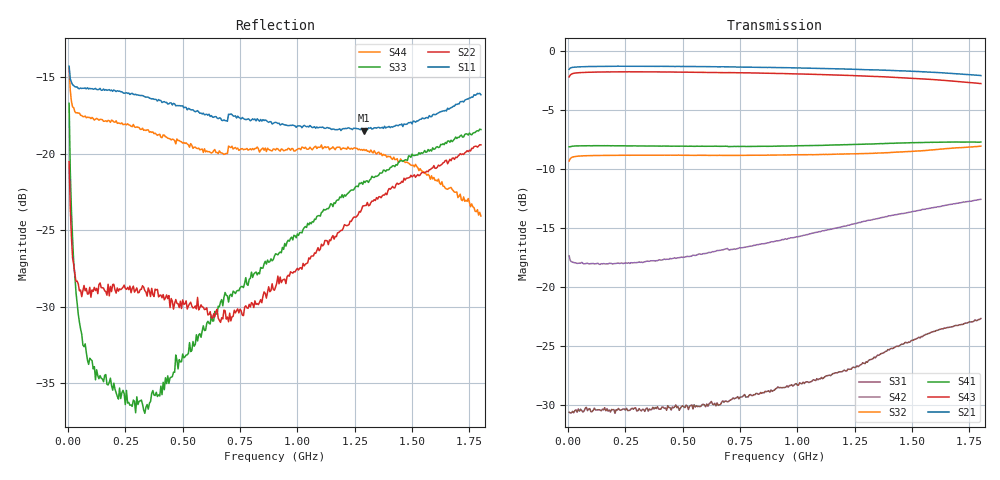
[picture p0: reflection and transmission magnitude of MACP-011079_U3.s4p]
!Agilent Technologies,E5071C,MY46110647,A.11.31
!Date: Tue Nov 07 14:18:09 2023
!Data & Calibration Information:
!MACP-011079 soldered onto PT-0003645 with F connectors, Calibration PT-0003653-TRL. Port1 (pin1) Port2 (pin6) Port3 (pin4) Port4 (pin3)
!Freq	S11:SOLT4(ON)	S12:SOLT4(ON)	S13:SOLT4(ON)	S14:SOLT4(ON)
!	S21:SOLT4(ON)	S22:SOLT4(ON)	S23:SOLT4(ON)	S24:SOLT4(ON)
!	S31:SOLT4(ON)	S32:SOLT4(ON)	S33:SOLT4(ON)	S34:SOLT4(ON)
!	S41:SOLT4(ON)	S42:SOLT4(ON)	S43:SOLT4(ON)	S44:SOLT4(ON)
!PortZ  Port1:75+j0  Port2:75+j0  Port3:75+j0  Port4:75+j0
!Above PortZ is port z conversion or system Z0 setting when saving the data.
!When reading, reference impedance value at option line is always used.
# Hz S MA R 75
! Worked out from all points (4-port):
!   360 points, 5 MHz to 1.8 GHz, reference 75 ohm
!   strongest paths, dB at 5 MHz, 455 MHz, 905 MHz, 1.355 GHz, 1.8 GHz:
!     S21: -1.6, -1.3, -1.4, -1.6, -2.1
!     S43: -2.2, -1.8, -1.9, -2.2, -2.8
!     S41: -8.1, -8.1, -8.1, -7.9, -7.7
!     S32: -9.3, -8.8, -8.8, -8.7, -8.1
!     S42: -17.4, -17.6, -16.1, -14.2, -12.6
!     S31: -30.6, -30.2, -28.6, -25.8, -22.7
!   lowest |S11| = -18.5 dB at 1.29 GHz (marker M1), VSWR 1.27, Z = 63.2 + j11.4 ohm
!   |S11| at or under -10 dB: start of sweep to end of sweep
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5000000  0.1931 161.8  0.8387 4.0  0.02866 20.8  0.3914 -177.7
         0.8365 4.0  0.09411 127.6  0.3431 9.1  0.1354 173.9
         0.02942 26.0  0.3417 9.0  0.1461 117.6  0.7741 7.3
         0.3925 -177.6  0.1354 173.6  0.7765 7.3  0.1914 150.3
2.5e7  0.1669 173.5  0.8537 0.6  0.02989 6.6  0.395 179.0
       0.8536 0.6  0.04333 151.8  0.3564 2.2  0.1279 176.8
       0.02925 5.9  0.356 2.2  0.04411 119.6  0.8039 1.4
       0.3949 179.1  0.1267 176.0  0.8042 1.3  0.1412 166.1
6.5e7  0.1637 176.2  0.8581 -1.1  0.02991 2.0  0.3963 175.8
       0.8579 -1.1  0.03565 175.4  0.3593 0.1  0.1265 175.8
       0.02946 0.6  0.3591 0.2  0.02369 132.1  0.8102 -1.3
       0.396 175.8  0.1258 174.9  0.8105 -1.3  0.1322 168.7
2.95e8  0.1563 170.7  0.8614 -7.9  0.02998 1.1  0.3956 159.5
        0.8615 -7.9  0.03578 -157.0  0.3615 -4.7  0.1306 164.2
        0.03068 -0.7  0.3617 -4.7  0.01423 113.2  0.8154 -10.9
        0.396 159.5  0.1266 162.8  0.8156 -10.9  0.1219 147.0
7.1e8  0.1348 156.1  0.8555 -19.7  0.03329 -0.0  0.3923 131.5
       0.8554 -19.7  0.0284 -126.4  0.3618 -11.6  0.1434 140.7
       0.0332 2.3  0.3609 -11.6  0.03471 50.0  0.8095 -27.1
       0.3934 131.6  0.1442 141.3  0.8094 -27.1  0.1047 94.9
1.29e9  0.1188 131.3  0.8321 -36.6  0.04151 1.7  0.4001 93.7
        0.8337 -36.6  0.06755 -101.3  0.368 -20.5  0.1834 106.3
        0.04743 4.3  0.3674 -20.2  0.08131 11.7  0.7827 -50.8
        0.4024 94.1  0.1897 104.5  0.7832 -50.9  0.1032 35.7
1.8e9  0.1558 116.9  0.7852 -52.3  0.06476 -9.1  0.4077 59.4
       0.7866 -52.5  0.1068 -125.3  0.3929 -28.7  0.2313 72.2
       0.07339 -9.7  0.3949 -28.6  0.1199 -13.7  0.7275 -74.0
       0.4112 59.6  0.235 69.3  0.7274 -74.0  0.06256 19.5
